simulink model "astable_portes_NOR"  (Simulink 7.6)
settings: Solver=ode15s  StartTime=0.0  StopTime=10  RelTol=1e-3
InitFcn:
  | clc
  | delete *.mat
StopFcn:
  | close all, clc
  | load es.mat
  | plot(x(1,:),x(2,:),x(1,:),x(3,:))
  | title('Sortie de l''astable et tension aux bornes de C')
  | xlabel('temps')
  | grid
libraries: fl_lib x5, nesl_utility x3, elec_lib x2

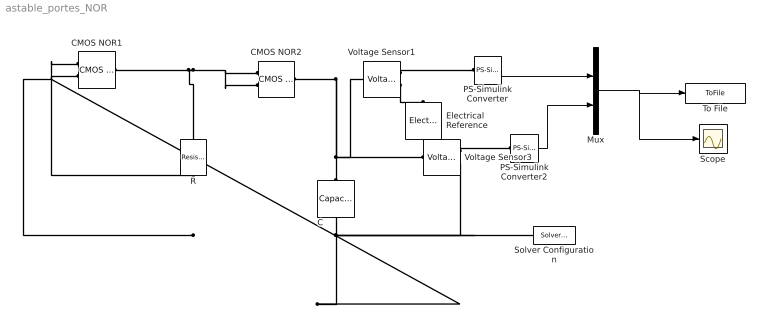
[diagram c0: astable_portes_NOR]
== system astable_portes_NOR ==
  C : fl_lib/Electrical/Electrical Elements/Capacitor  DialogController=NetworkEngine.DynNeDlgSource  SystemSampleTime=-1  c=1e-3 F  v0=0 V  r=1e-6 Ohm  g=0 1/Ohm  i_Log=off  v_Log=off  vc_Log=off  LocalVarNames=|i|v|vc  LocalVarDescs=|i|v|Internal variable for voltage across capacitor term  LocalVarLogging=[0 0 0]
  CMOS NOR1 : elec_lib/Integrated Circuits/Logic/CMOS NOR  DialogController=NetworkEngine.DynNeDlgSource  SystemSampleTime=-1  V_IL=2 V  V_IH=3 V  C_IN=5 pF  output_type=1  V_OL=0 V  V_OH=5 V  V_CC=5 V  V_meas=5 V  R_OUT=25 Ohm  R_OH=[ 25 250 ] Ohm  I_OH=63 mA  R_OL=[ 30 800 ] Ohm  I_OL=-45 mA  Delay=25 ns  Ron=5 Ohm  Vf=0.6 V  output_state=1  LocalVarLogging=[]
  CMOS NOR2 : elec_lib/Integrated Circuits/Logic/CMOS NOR  DialogController=NetworkEngine.DynNeDlgSource  SystemSampleTime=-1  V_IL=2 V  V_IH=3 V  C_IN=5 pF  output_type=1  V_OL=0 V  V_OH=5 V  V_CC=5 V  V_meas=5 V  R_OUT=25 Ohm  R_OH=[ 25 250 ] Ohm  I_OH=63 mA  R_OL=[ 30 800 ] Ohm  I_OL=-45 mA  Delay=25 ns  Ron=5 Ohm  Vf=0.6 V  output_state=1  LocalVarLogging=[]
  Electrical Reference : fl_lib/Electrical/Electrical Elements/Electrical Reference  DialogController=NetworkEngine.DynNeDlgSource  SystemSampleTime=-1  i_Log=off  LocalVarNames=|i  LocalVarDescs=|i  LocalVarLogging=0
  Mux : Mux  Inputs=2
  PS-Simulink Converter : nesl_utility/PS-Simulink Converter  DialogController=NetworkEngine.DynNeUtilDlgSource  SystemSampleTime=-1  PhysicalDomain=network_engine_domain  LeftPortType=input  RightPortType=output  SubClassName=ps_output  Unit=1  AffineConversion=off
  PS-Simulink Converter2 : nesl_utility/PS-Simulink Converter  DialogController=NetworkEngine.DynNeUtilDlgSource  SystemSampleTime=-1  PhysicalDomain=network_engine_domain  LeftPortType=input  RightPortType=output  SubClassName=ps_output  Unit=1  AffineConversion=off
  R : fl_lib/Electrical/Electrical Elements/Resistor  DialogController=NetworkEngine.DynNeDlgSource  SystemSampleTime=-1  R=1.2 kOhm  i_Log=off  v_Log=off  LocalVarNames=|i|v  LocalVarDescs=|i|v  LocalVarLogging=[0 0]
  Scope : Scope
  Solver Configuration : nesl_utility/Solver Configuration  DialogController=NetworkEngine.DynNeUtilDlgSource  SystemSampleTime=-1  PhysicalDomain=network_engine_domain  LeftPortType=input  RightPortType=generic  SubClassName=solver  Accelerate=off  Profile=off  ResidualTolerance=1e-9  MaxNonlinIter=12  MaxModeIter=2  DoFixedCost=off  UseLocalSampling=off  DoDC=off  LinearAlgebra=Sparse  LocalSolverSampleTime=.001  LocalSolverChoice=NE_BACKWARD_EULER_ADVANCER  UseLocalSolver=off
  To File : ToFile  Filename=es.mat  MatrixName=x
  Voltage Sensor1 : fl_lib/Electrical/Electrical Sensors/Voltage Sensor  DialogController=NetworkEngine.DynNeDlgSource  SystemSampleTime=-1  i1_Log=off  v1_Log=off  LocalVarNames=|i1|v1  LocalVarDescs=|i1|v1  LocalVarLogging=[]
  Voltage Sensor3 : fl_lib/Electrical/Electrical Sensors/Voltage Sensor  DialogController=NetworkEngine.DynNeDlgSource  SystemSampleTime=-1  i1_Log=off  v1_Log=off  LocalVarNames=|i1|v1  LocalVarDescs=|i1|v1  LocalVarLogging=[]
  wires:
  Mux/1 -> To File/1, Scope/1
  PS-Simulink Converter/1 -> Mux/1
  PS-Simulink Converter2/1 -> Mux/2
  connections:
  Voltage Sensor1/RConn1 -- PS-Simulink Converter/LConn1
  CMOS NOR2/LConn1 -- CMOS NOR2/LConn2 -- CMOS NOR1/RConn1 -- R/RConn1
  Voltage Sensor1/LConn1 -- CMOS NOR2/RConn1 -- C/LConn1 -- Voltage Sensor3/LConn1
  Voltage Sensor1/RConn2 -- Electrical Reference/LConn1
  Voltage Sensor3/RConn1 -- PS-Simulink Converter2/LConn1
  C/RConn1 -- Solver Configuration/RConn1 -- Voltage Sensor3/RConn2 -- R/LConn1 -- CMOS NOR1/LConn2 -- CMOS NOR1/LConn1
